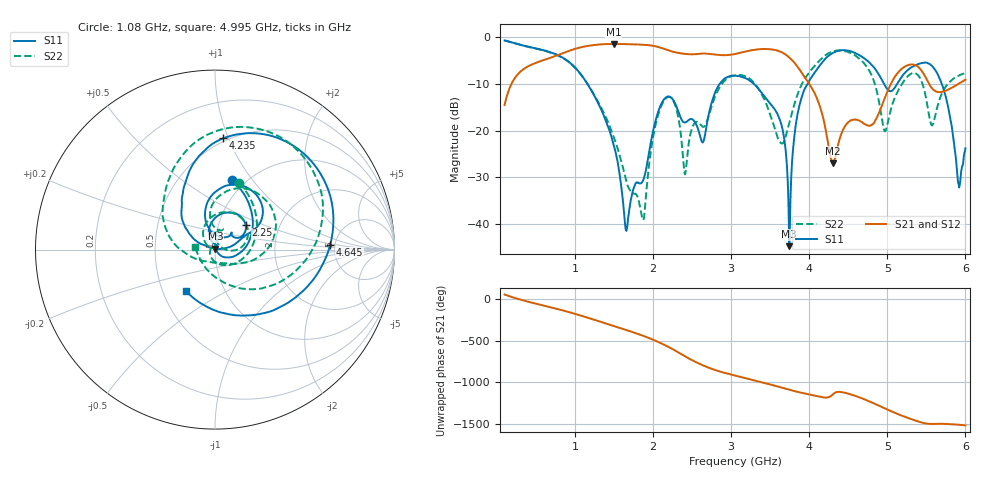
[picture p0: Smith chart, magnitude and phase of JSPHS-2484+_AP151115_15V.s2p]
!Mini-Circuits Laboratory
!S-Parameters
!Run/Lot/Date Code:MF33450/NA/1551
!Fixture/SN/Due: 90-4-20-21/70546/03/17/16
!Connection:PORT<IN> - pin<1>; PORT<OUT> - pin<7>;PORT<BIAS> - pin<4>;
!Tested With:PORT EXTENTION
!Network Analyzer:AG E5071C/74883/05/12/16
!Created: 01-07-2016 at 14:11:36
!MODEL: JSPHS-2484+
!S/N: V=15V
# MHZ S DB R 50
!Frequency  S11 dB  S11 DEG  S21 dB  S21 DEG  S12 dB  S12 DEG  S22 dB  S22 DEG
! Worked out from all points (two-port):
!   1181 points, 100 MHz to 6 GHz, reference 50 ohm
!   highest |S21| = -1.41 dB at 1.5 GHz (marker M1); lowest = -27.0 dB at 4.3 GHz (marker M2)
!   |S21| within 3 dB of the highest: 681.9 MHz to 3.751 GHz (3.069 GHz wide, 138 % of centre)
!   lowest |S11| = -44.8 dB at 3.745 GHz (marker M3), VSWR 1.01, Z = 50.2 + j0.537 ohm
!   |S11| at or under -10 dB: 1.162 GHz to 2.853 GHz (1.691 GHz wide, 84.3 % of centre); 3.293 GHz to 3.978 GHz (685 MHz wide, 18.8 % of centre); 5.698 GHz to end of sweep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
!   |S22| runs from -39.1 to -0.7 dB; largest |S21 - S12| = 0.0065
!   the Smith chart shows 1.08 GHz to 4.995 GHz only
!   S11 on the Smith chart (normalised r, x): 1.08 GHz: 0.87, +0.80; 2.25 GHz: 1.35, +0.39; 4.235 GHz: 0.47, +0.96; 4.645 GHz: 4.55, +0.44; 4.995 GHz: 0.66, -0.33
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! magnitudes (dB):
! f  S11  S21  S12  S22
! 100 MHz  -0.7  -14.5  -14.5  -0.7
! 1.08 GHz  -8.0  -2.1  -2.1  -8.1
! 1.085 GHz  -8.1  -2.1  -2.1  -8.2
! 1.5 GHz  -23.3  -1.4  -1.4  -21.4
! 1.655 GHz  -41.4  -1.5  -1.4  -30.7
! 1.87 GHz  -30.8  -1.6  -1.6  -39.1
! 2.07 GHz  -15.8  -2.1  -2.1  -16.4
! 2.25 GHz  -13.2  -3.1  -3.1  -13.3
! 2.41 GHz  -18.2  -3.5  -3.5  -29.4
! 3.05 GHz  -8.2  -3.6  -3.6  -8.1
! 3.605 GHz  -16.9  -2.9  -2.9  -21.8
! 3.745 GHz  -44.8  -4.3  -4.3  -18.3
! 4.035 GHz  -8.4  -10.9  -11.0  -6.8
! 4.235 GHz  -4.1  -22.0  -21.9  -3.5
! 4.3 GHz  -3.4  -27.0  -27.0  -3.0
! 4.645 GHz  -3.8  -17.9  -17.8  -4.6
! 4.995 GHz  -11.0  -11.9  -11.8  -19.1
! 5.02 GHz  -11.4  -10.9  -10.9  -17.2
! 5.345 GHz  -6.1  -5.9  -5.9  -7.6
! 5.555 GHz  -5.9  -10.5  -10.5  -18.3
! 5.915 GHz  -31.6  -9.9  -9.9  -8.2
! 6 GHz  -23.8  -9.1  -9.1  -7.7
